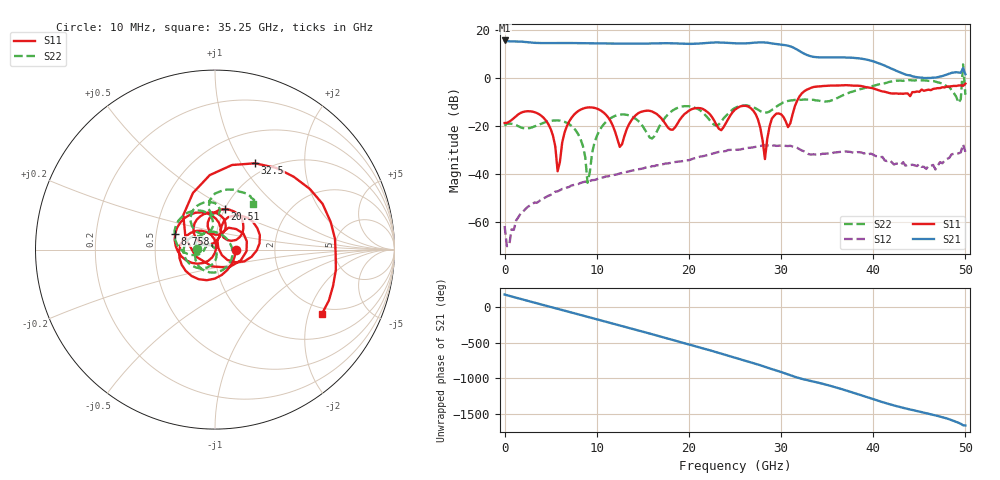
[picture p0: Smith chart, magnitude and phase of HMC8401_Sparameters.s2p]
! Analog Devices Inc.
! Device:  HMC8401
! Description: GaAs PHEMPT Low Noise Amplifier
! Frequency:  0.00 -  28.00 GHz
! Die Size: 2.55mmx1.5mmx0.05mm
! Conditions:	TA = 25degC, VDD = 7.5 V, IDQ = 60 mA, VGG2 = open, unless otherwise stated. When using VGG2, it is recommended to limit VGG2 from -2 V to +2.6 V
!		Note: Adjust the VGG1 supply voltage between -2 V and 0 V to achieve IDQ = 60 mA typical.
! Misc:JM
! Freq(GHz)	S11a(dB)	S11p(deg)	S21a(dB)	S21p(deg)	S12a(dB)	S12p(deg)	S22a(dB)	S22p(deg)
# GHz S  dB  R 50
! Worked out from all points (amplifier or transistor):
!   201 points, 10 MHz to 50 GHz, reference 50 ohm
!   highest |S21| = 15.7 dB at 10 MHz (marker M1)
!   |S21| within 3 dB of that: start of sweep to 31.35 GHz
!   unconditionally stable (mu >= 1): start of sweep to 49.67 GHz; 49.85744 GHz to end of sweep
!   at 8.258 GHz: K = 13.64, MAG = 14.8 dB, |S12| = -43.7 dB
!   at 25.01 GHz: K = 2.78, MAG = 14.9 dB, |S12| = -29.9 dB
!   at 50 GHz: K = 4.35, MAG = 6.9 dB, |S12| = -30.8 dB
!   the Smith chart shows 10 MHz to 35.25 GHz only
!   S11 on the Smith chart (normalised r, x): 10 MHz: 1.26, -0.01; 8.758 GHz: 0.63, +0.12; 20.51 GHz: 1.00, +0.48; 32.5 GHz: 0.86, +1.15; 35.25 GHz: 1.78, -2.46
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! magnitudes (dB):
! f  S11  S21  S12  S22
! 10 MHz  -18.7  15.7  -61.7  -19.9
! 509.9 MHz  -18.2  15.4  -69.8  -19.0
! 4.259 GHz  -16.6  14.6  -50.1  -18.6
! 5.759 GHz  -38.9  14.6  -47.3  -17.6
! 8.508 GHz  -12.7  14.6  -43.4  -28.4
! 8.758 GHz  -12.4  14.5  -43.2  -33.0
! 9.008 GHz  -12.3  14.5  -43.3  -43.7
! 10.26 GHz  -13.1  14.5  -41.7  -22.1
! 12.51 GHz  -28.7  14.4  -39.8  -15.2
! 16.76 GHz  -15.8  14.5  -36.4  -20.5
! 20.51 GHz  -12.7  14.3  -33.5  -12.1
! 25.01 GHz  -13.2  14.5  -29.9  -12.5
! 27.25 GHz  -15.1  14.8  -28.7  -12.6
! 28.25 GHz  -33.8  14.9  -28.0  -14.3
! 29 GHz  -16.9  14.5  -28.4  -13.3
! 32.5 GHz  -5.5  10.2  -30.5  -8.9
! 33.5 GHz  -3.7  8.9  -31.8  -9.0
! 35.25 GHz  -3.2  8.7  -31.5  -9.6
! 41.75 GHz  -6.2  4.4  -34.3  -1.5
! 49.25 GHz  -3.1  2.4  -31.4  -10.3
! 49.75 GHz  -3.2  4.1  -27.7  5.7
! 50 GHz  -2.3  1.6  -30.8  -7.0
